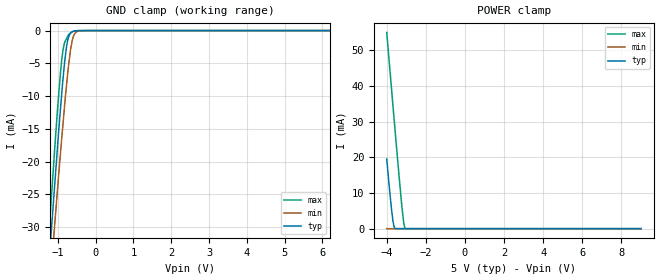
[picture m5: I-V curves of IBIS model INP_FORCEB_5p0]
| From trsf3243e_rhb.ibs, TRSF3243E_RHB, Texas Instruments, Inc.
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[Model]   INP_FORCEB_5p0
Model_type   Input
Vinl = 0.8
Vinh = 2.4
|   typ   min   max
C_comp   0.748pF	0.718pF	0.787pF
[Voltage Range]   5   4.5   5.5
[Temperature Range]   27   110   -40
[Power Clamp Reference]   5   4.5   5.5
[GND Clamp Reference]   0   0   0
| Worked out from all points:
|   GND clamp passes 1 mA (typ) near -0.71 V on its own axis
|   POWER clamp passes 1 mA (typ) near -3.64 V on its own axis
[GND Clamp]
|   Voltage   I(typ)   I(min)   I(max)
-4V       -268.4mA   -254.7mA   -282.4mA
-1.341V   -44.12mA   -48.73mA   -40.42mA
-1.22V    -34.23mA   -39.62mA   -29.65mA
-1.179V   -31.04mA   -36.55mA   -26.13mA
-1.072V   -22.72mA   -28.84mA   -17.14mA
-894.1mV  -9.453mA   -16.24mA   -4.329mA
-819.8mV  -4.816mA   -11.39mA   -1.777mA
-745.9mV  -1.667mA   -6.963mA   -952.3uA
-667.2mV  -425.8uA   -3.059mA   -358.6uA
-603.6mV  -151.3uA   -1.203mA   -132.2uA
-411.9mV  -10.73uA   -21.66uA   -3.311uA
9V        0A         0A         0A
[POWER Clamp]
|   Voltage   I(typ)   I(min)   I(max)
-4V       19.5mA     4.956uA    54.98mA
-3.859V   11.1mA     51.91nA    45.82mA
-3.745V   4.891mA    27.69nA    38.47mA
-3.685V   2.243mA    14.94nA    34.62mA
-3.639V   851.2uA    5.172nA    31.67mA
-3.548V   40.18uA    0A         25.88mA
-3.387V   153.5nA    0A         15.76mA
-3.229V   17.59nA    0A         6.473mA
-3.14V    3.207nA    0A         2.064mA
-3.107V   0A         0A         912.6uA
-3.053V   0A         0A         113.7uA
9V        0A         0A         0A
